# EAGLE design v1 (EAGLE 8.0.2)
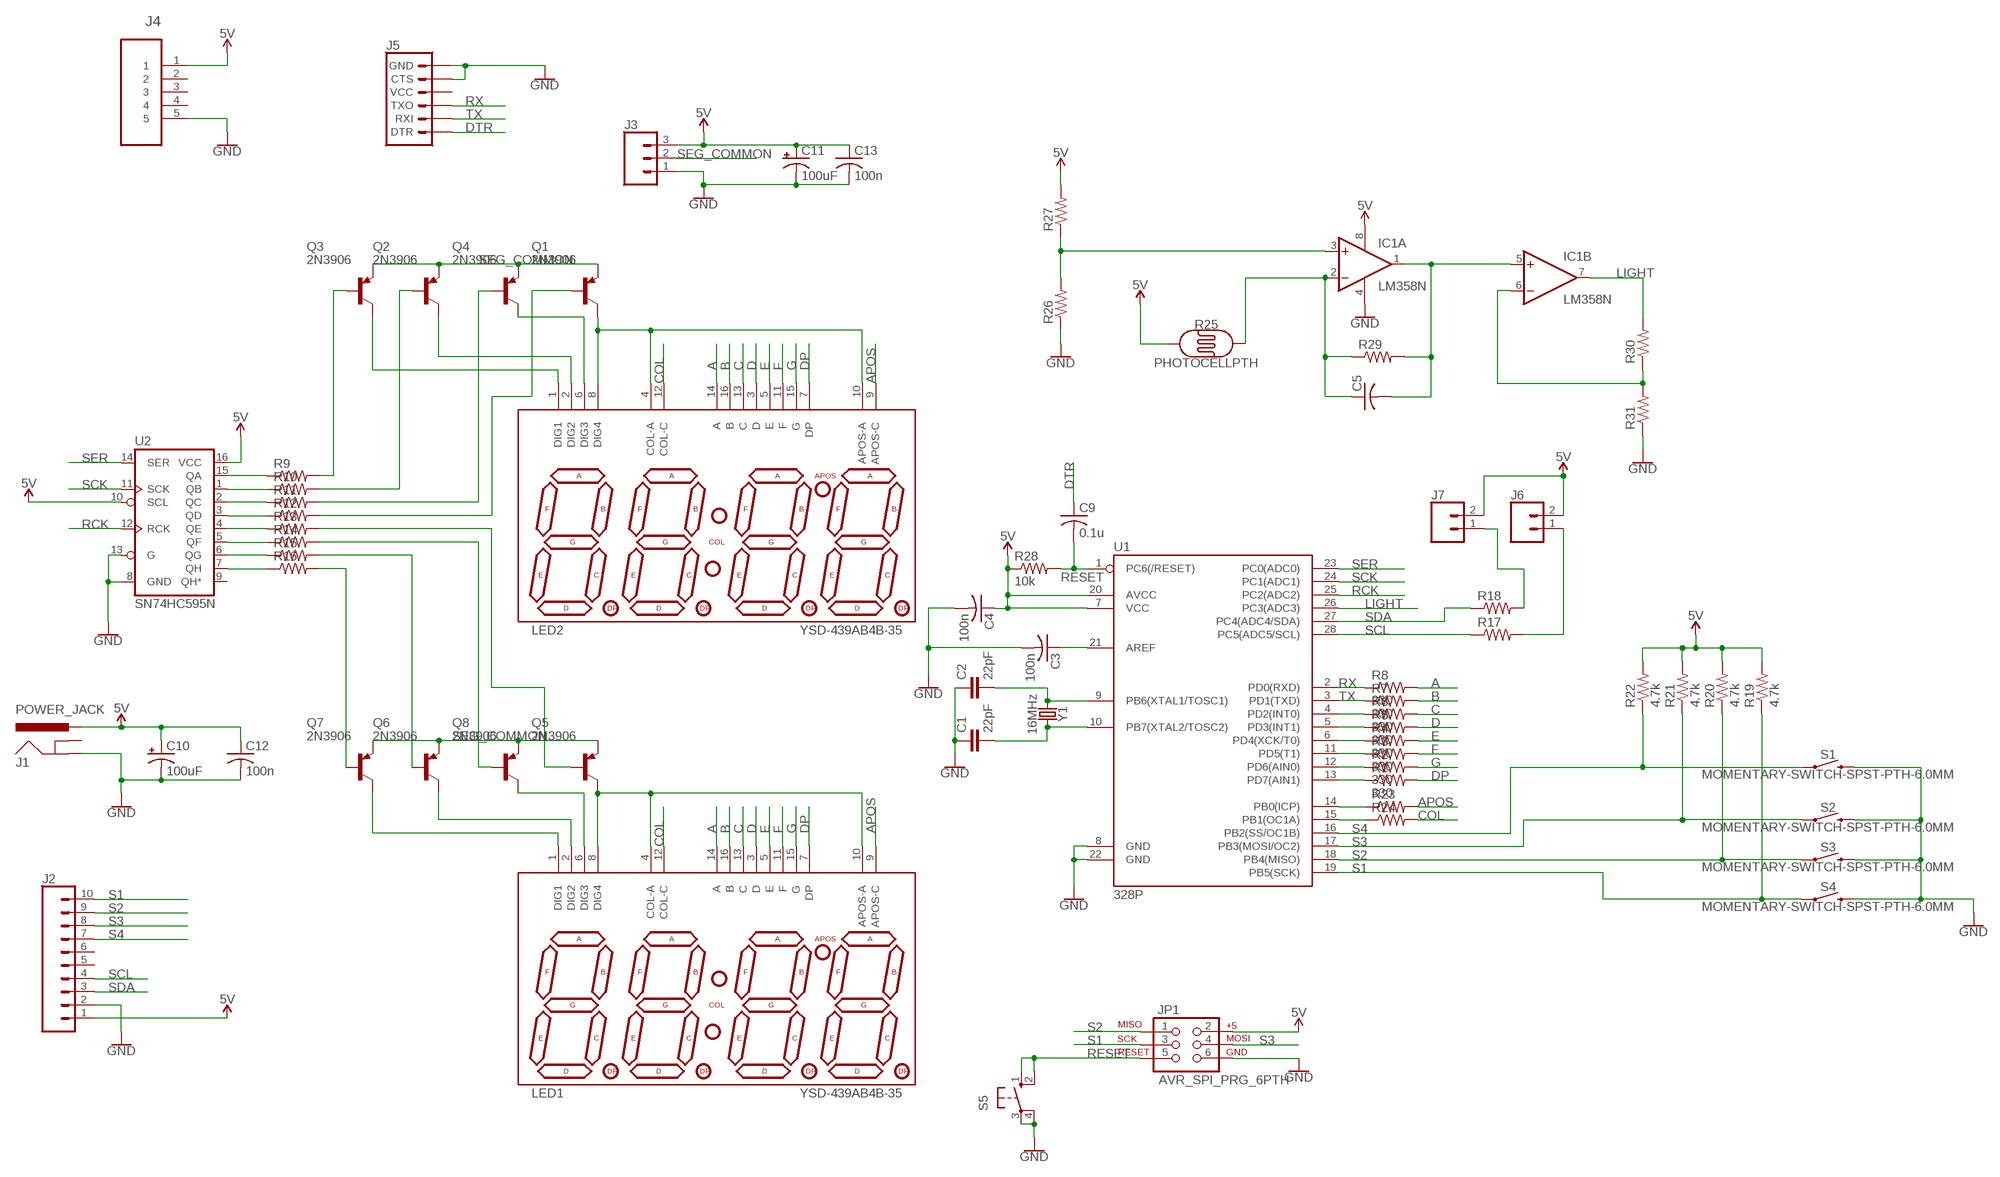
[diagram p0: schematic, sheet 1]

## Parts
C1  22pF  22PF-PTH-2.54MM-200V-5%  [CAP-PTH-2.54]
C2  22pF  22PF-PTH-2.54MM-200V-5%  [CAP-PTH-2.54]
C3  100n  C-US025-025X050  [C025-025X050]
C4  100n  C-US025-025X050  [C025-025X050]
C5  C-US025-025X050  [C025-025X050]
C9  0.1u  C-US025-025X050  [C025-025X050]
C10  100uF  100UF-POLAR-RADIAL-2.5MM-25V-20%  [CPOL-RADIAL-2.5MM-6.5MM]
C11  100uF  100UF-POLAR-RADIAL-2.5MM-25V-20%  [CPOL-RADIAL-2.5MM-6.5MM]
C12  100n  C-US025-025X050  [C025-025X050]
C13  100n  C-US025-025X050  [C025-025X050]
IC1  LM358N  [DIL08]
J1  POWER_JACK  [POWER_JACK_PTH]
J2  CONN_10"  [1X10]
J3  CONN_03  [1X03]
J4  47346-0001  [MOLEX_47346-0001]
J5  6_PIN_SERIAL_TARGET  [1X06]
J6  CONN_02  [1X02]
J7  CONN_02  [1X02]
JP1  AVR_SPI_PRG_6PTH  [2X3]
LED1  YSD-439AB4B-35  7-SEGMENT-4DIGIT-10MM-BLUE  [7-SEGMENT-4DIGIT-YOUNGSUN]
LED2  YSD-439AB4B-35  7-SEGMENT-4DIGIT-10MM-BLUE  [7-SEGMENT-4DIGIT-YOUNGSUN]
Q1  2N3906  [TO92]
Q2  2N3906  [TO92]
Q3  2N3906  [TO92]
Q4  2N3906  [TO92]
Q5  2N3906  [TO92]
Q6  2N3906  [TO92]
Q7  2N3906  [TO92]
Q8  2N3906  [TO92]
R1  330  R-US_0204/5  [0204/5]
R2  330  R-US_0204/5  [0204/5]
R3  330  R-US_0204/5  [0204/5]
R4  330  R-US_0204/5  [0204/5]
R5  330  R-US_0204/5  [0204/5]
R6  330  R-US_0204/5  [0204/5]
R7  330  R-US_0204/5  [0204/5]
R8  330  R-US_0204/5  [0204/5]
R9  R-US_0204/5  [0204/5]
R10  R-US_0204/5  [0204/5]
R11  R-US_0204/5  [0204/5]
R12  R-US_0204/5  [0204/5]
R13  R-US_0204/5  [0204/5]
R14  R-US_0204/5  [0204/5]
R15  R-US_0204/5  [0204/5]
R16  R-US_0204/5  [0204/5]
R17  R-US_0204/5  [0204/5]
R18  R-US_0204/5  [0204/5]
R19  4.7k  R-US_0204/5  [0204/5]
R20  4.7k  R-US_0204/5  [0204/5]
R21  4.7k  R-US_0204/5  [0204/5]
R22  4.7k  R-US_0204/5  [0204/5]
R23  R-US_0204/5  [0204/5]
R24  R-US_0204/5  [0204/5]
R25  PHOTOCELLPTH  [PHOTOCELL]
R26  R-US_0204/5  [0204/5]
R27  R-US_0204/5  [0204/5]
R28  10k  R-US_0204/5  [0204/5]
R29  R-US_0204/5  [0204/5]
R30  R-US_0204/5  [0204/5]
R31  R-US_0204/5  [0204/5]
S1  MOMENTARY-SWITCH-SPST-PTH-6.0MM  [TACTILE_SWITCH_PTH_6.0MM]
S2  MOMENTARY-SWITCH-SPST-PTH-6.0MM  [TACTILE_SWITCH_PTH_6.0MM]
S3  MOMENTARY-SWITCH-SPST-PTH-6.0MM  [TACTILE_SWITCH_PTH_6.0MM]
S4  MOMENTARY-SWITCH-SPST-PTH-6.0MM  [TACTILE_SWITCH_PTH_6.0MM]
S5  10-XX  [B3F-10XX]
U1  328P  ATMEGA328P_PDIP  [DIP28]
U2  SN74HC595N  74HC595N  [DIP16]
Y1  16MHz  CRYSTAL-16MHZPTH-HC49US  [HC49US]

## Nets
5V [SUPPLY]: C4.1 C10.1(+) C11.1(+) C12.1 C13.1 IC1.8(P:V+) J1.PWR J2.1 J3.3 J4.1 J6.2 J7.2 JP1.2 R19.2 R20.2 R21.2 R22.2 R25.1 R27.2 R28.1 U1.7(VCC) U1.20(AVCC) U2.10(SCL) U2.16(VCC)
A: LED1.14(A) LED2.14(A) R8.2
APOS: LED1.9(APOS-C) LED2.9(APOS-C) R23.2
B: LED1.16(B) LED2.16(B) R7.2
C: LED1.13(C) LED2.13(C) R6.2
COL: LED1.12(COL-C) LED2.12(COL-C) R24.2
D: LED1.3(D) LED2.3(D) R5.2
DP: LED1.7(DP) LED2.7(DP) R1.2
DTR: C9.1 J5.1(DTR)
E: LED1.5(E) LED2.5(E) R4.2
F: LED1.11(F) LED2.11(F) R3.2
G: LED1.15(G) LED2.15(G) R2.2
GND [SUPPLY]: C1.1 C2.1 C3.2 C4.2 C10.2(-) C11.2(-) C12.2 C13.2 IC1.4(P:V-) J1.GND J2.2 J3.1 J4.5 J5.5(CTS) J5.6(GND) JP1.6 R26.1 R31.1 S1.3 S2.3 S3.3 S4.3 S5.3(P) S5.4(P1) U1.8(GND) U1.22(GND) U2.8(GND) U2.13(G)
LIGHT: IC1.7(B:OUT) R30.2 U1.26(PC3(ADC3))
N$2: R24.1 U1.15(PB1(OC1A))
N$3: R6.1 U1.4(PD2(INT0))
N$4: R5.1 U1.5(PD3(INT1))
N$5: R4.1 U1.6(PD4(XCK/T0))
N$6: R3.1 U1.11(PD5(T1))
N$7: R2.1 U1.12(PD6(AIN0))
N$8: R1.1 U1.13(PD7(AIN1))
N$9: C2.2 U1.9(PB6(XTAL1/TOSC1)) Y1.1
N$10: C1.2 U1.10(PB7(XTAL2/TOSC2)) Y1.2
N$11: LED2.4(COL-A) LED2.8(DIG4) LED2.10(APOS-A) Q1.1(C)
N$12: LED2.6(DIG3) Q4.1(C)
N$13: LED2.2(DIG2) Q2.1(C)
N$14: LED2.1(DIG1) Q3.1(C)
N$15: LED1.4(COL-A) LED1.8(DIG4) LED1.10(APOS-A) Q5.1(C)
N$16: IC1.3(A:+IN) R26.2 R27.1
N$17: LED1.6(DIG3) Q8.1(C)
N$18: LED1.2(DIG2) Q6.1(C)
N$19: C5.1 IC1.2(A:-IN) R25.2 R29.1
N$20: LED1.1(DIG1) Q7.1(C)
N$21: Q3.2(B) R9.2
N$22: Q2.2(B) R10.2
N$23: Q4.2(B) R11.2
N$24: Q1.2(B) R12.2
N$25: Q5.2(B) R13.2
N$26: Q8.2(B) R14.2
N$27: Q6.2(B) R15.2
N$28: Q7.2(B) R16.2
N$29: R9.1 U2.15(QA)
N$30: R10.1 U2.1(QB)
N$31: R11.1 U2.2(QC)
N$32: R12.1 U2.3(QD)
N$33: R13.1 U2.4(QE)
N$34: R14.1 U2.5(QF)
N$35: R15.1 U2.6(QG)
N$36: R16.1 U2.7(QH)
N$37: C3.1 U1.21(AREF)
N$38: C5.2 IC1.1(A:OUT) IC1.5(B:+IN) R29.2
N$39: J7.1 R18.2
N$40: J6.1 R17.2
N$43: IC1.6(B:-IN) R30.1 R31.2
N$46: R23.1 U1.14(PB0(ICP))
RCK: U1.25(PC2(ADC2)) U2.12(RCK)
RESET: C9.2 JP1.5 R28.2 S5.1(S) S5.2(S1) U1.1(PC6(/RESET))
RX: J5.3(TXO) R8.1 U1.2(PD0(RXD))
S1: J2.10 JP1.3 R19.1 S4.1 U1.19(PB5(SCK))
S2: J2.9 JP1.1 R20.1 S3.1 U1.18(PB4(MISO))
S3: J2.8 JP1.4 R21.1 S2.1 U1.17(PB3(MOSI/OC2))
S4: J2.7 R22.1 S1.1 U1.16(PB2(SS/OC1B))
SCK: U1.24(PC1(ADC1)) U2.11(SCK)
SCL: J2.4 R17.1 U1.28(PC5(ADC5/SCL))
SDA: J2.3 R18.1 U1.27(PC4(ADC4/SDA))
SEG_COMMON [SUPPLY]: J3.2 Q1.3(E) Q2.3(E) Q3.3(E) Q4.3(E) Q5.3(E) Q6.3(E) Q7.3(E) Q8.3(E)
SER: U1.23(PC0(ADC0)) U2.14(SER)
TX: J5.2(RXI) R7.1 U1.3(PD1(TXD))
Unconnected: J1.GNDBREAK J2.5 J2.6 J4.2 J4.3 J4.4 J5.4(VCC) U2.9(QH*)

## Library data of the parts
C1 C2 = SparkFun-Capacitors:22PF: 22pF ceramic capacitors; PROD_ID: CAP-09128
C3-C5 C9 C12 C13 = adafruit:C-US: CAPACITOR, American symbol
C10 C11 = SparkFun-Capacitors:100UF-POLAR: 100µF polarized capacitors; PROD_ID: CAP-08439
IC1 = linear:LM358: OP AMP also LM158; LM258; LM2904 Source: http://cache.national.com/ds/LM/LM158.pdf
J1 = SparkFun-Connectors:POWER_JACK: Power Jack Connector This is the standard 5.5mm barrel jack for power. The PTH is the most common, proven, reliable, footprint. The Slot footprint only works if the mill layer is transmitted to the PCB fab house so be warned. Here are the connectors we sell at SparkFun: DC Barrel Power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; PROD_ID: CONN-08197
J2 = SparkFun-Connectors:CONN_10: Multi connection point. Often used as Generic Header-pin footprint for 0.1 inch spaced/style header connections On any of the 0.1 inch spaced packages, you can populate with these: Break Away Headers - Straight (PRT-00116) Break Away Male Headers - Right Angle (PRT-00553) Female Headers (PRT-00115)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; PROD_ID: CONN-11563
J3 = SparkFun-Connectors:CONN_03: Multi connection point. Often used as Generic Header-pin footprint for 0.1 inch spaced/style header connections On any of the 0.1 inch spaced packages, you can populate with these: Break Away Headers - Straight (PRT-00116) Break Away Male Headers - Right Angle (PRT-00553) Female Headers (PRT-00115)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
J4 = Molex-47346-0001:47346-0001: CONN RCPT 5POS MICRO USB R/A SMD; MPN: 47346-0001; OC_FARNELL: 1568026; OC_NEWARK: 47M0505; PACKAGE: 5 POS MICRO USB R/A; SUPPLIER: MOLEX
J5 = SparkFun-Connectors:6_PIN_SERIAL_TARGET: 6-pin header connection for use with the "FTDI BASIC" pinout - TARGET SIDE. Also known as "Arduino Serial Program Header". It is used to mate with our FTDI Basic serial programmers using the Arduino IDE. Note, this device has "TARGET" in the name. It is intended to be used on a design that contains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
J6 J7 = SparkFun-Connectors:CONN_02: Multi connection point. Often used as Generic Header-pin footprint for 0.1 inch spaced/style header connections
JP1 = SparkFun-Connectors:AVR_SPI_PRG_6: AVR ISP 6 Pin This is the reduced ISP connector for AVR programming. Common on Arduino. This footprint will take up less PCB space and can be used with a 10-pin to 6-pin adapter such as SKU: BOB-08508 **Special note about "TEST_POINT" package. The stop mask is on the top side, so if you want your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
LED1 LED2 = SparkFun-LED:7-SEGMENT-4DIGIT-10MM: 4 Digit 7 Segment Display This is a part for the 4-Digit 7-segment LEDs from Young Sun. Different from the Digikey LEDs, all 16 pins are used. The LONGPADS Variant is used for a test jig, but you may like it because there is more pad to solder to. If you are concerned about routing space, the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; PROD_ID: COMP-09664
Q1-Q8 = transistor-pnp:2N3906: PNP Transistor
R1-R24 R26-R31 = rcl:R-US_: RESISTOR, American symbol
R25 = SparkFun-Sensors:PHOTOCELL: Photocell (Photodetector, Photo Resistor, CdS); PROD_ID: COMP-09129; SF_ID: SEN-09088
S1-S4 = SparkFun-Switches:MOMENTARY-SWITCH-SPST: Momentary Switch (Pushbutton) - SPST; PROD_ID: SWCH-08441; SF_SKU: COM-00097
S5 = switch-omron:10-XX: OMRON SWITCH; MPN: B3F-1000; OC_FARNELL: 176432; OC_NEWARK: 36M3542
U1 = SparkFun-IC-Microcontroller:ATMEGA328P_PDIP: Atmel 328P Through hole ATMEGA328P uC used in the Arduino 32kb flash, 1k EEPROM, 2k SRAM Datasheet SparkFun Products Storefront component: AVR 28 Pin 20MHz 32K 6A/D - ATMega328P (COM-09061) SparkFun Simon Says - Through-Hole Soldering Kit (KIT-10547) SparkFun Learn to Solder - Simon Says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; PROD_ID: IC-09136
U2 = SparkFun-IC-Logic:74*595: 8-Bit Shift Register (Serial to Parallel) Datasheet SparkFun Products SparkFun Shift Register Breakout - 74HC595 (BOB-10680); PROD_ID: IC-13123
Y1 = SparkFun-Clocks:CRYSTAL-16MHZ: 16MHz Crystal; PROD_ID: XTAL-08181; SF_ID: COM-00536

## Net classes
0 default: width 0.254 mm, drill 0.356 mm, clearance 0.2 mm
1 SUPPLY: width 0.4 mm, drill 0.4 mm, clearance 0.2 mm to class 0, clearance 0.2 mm

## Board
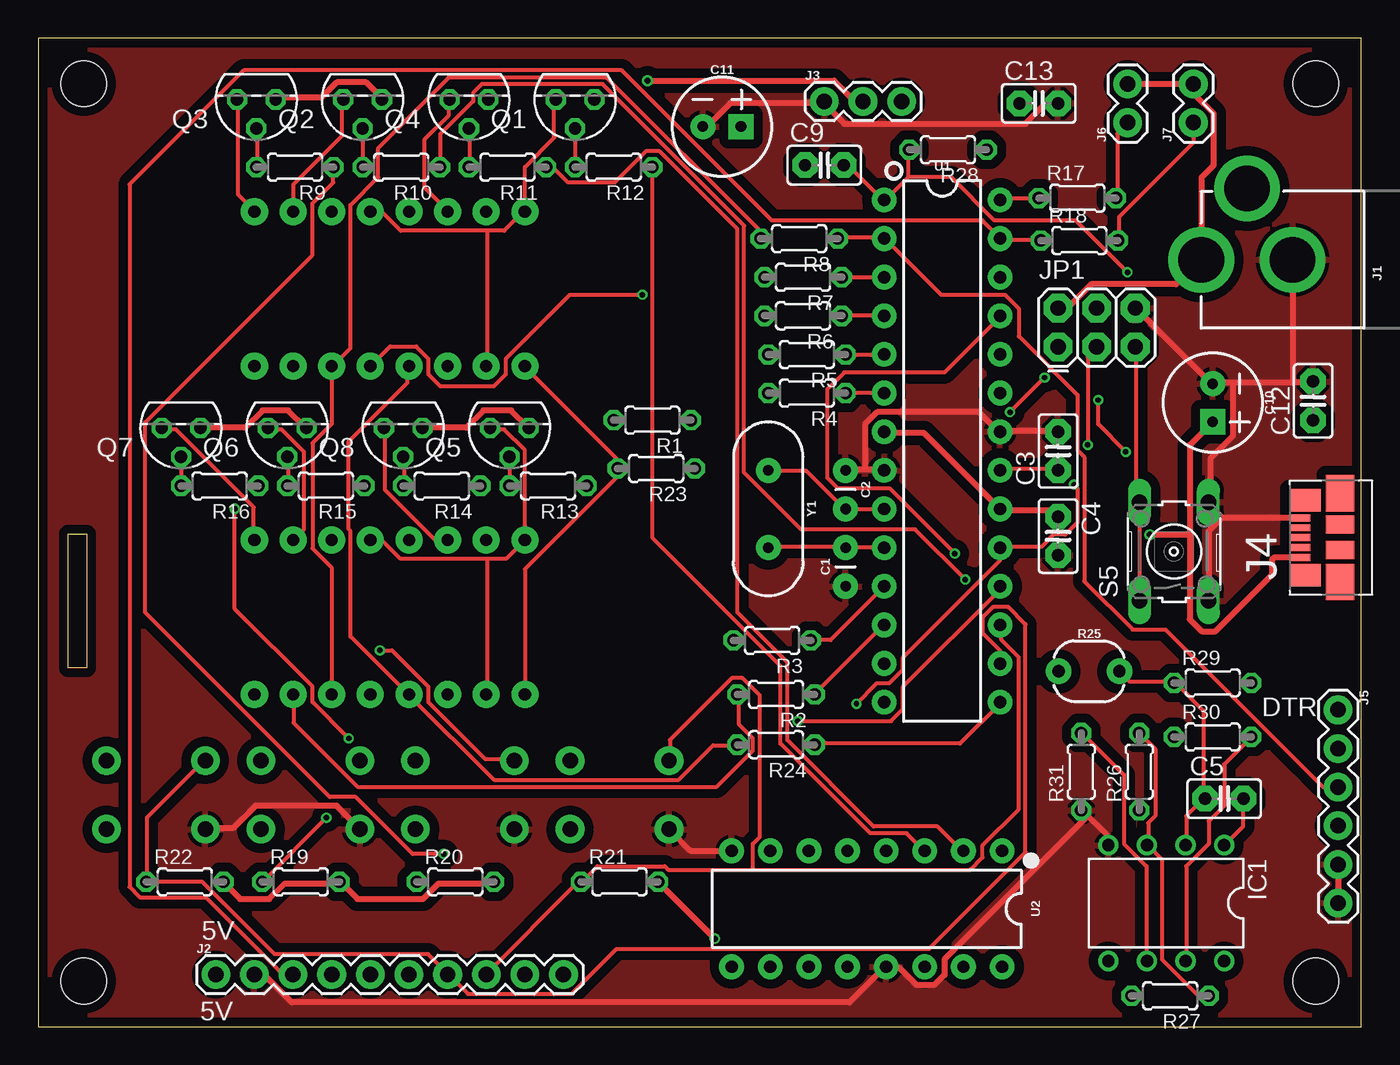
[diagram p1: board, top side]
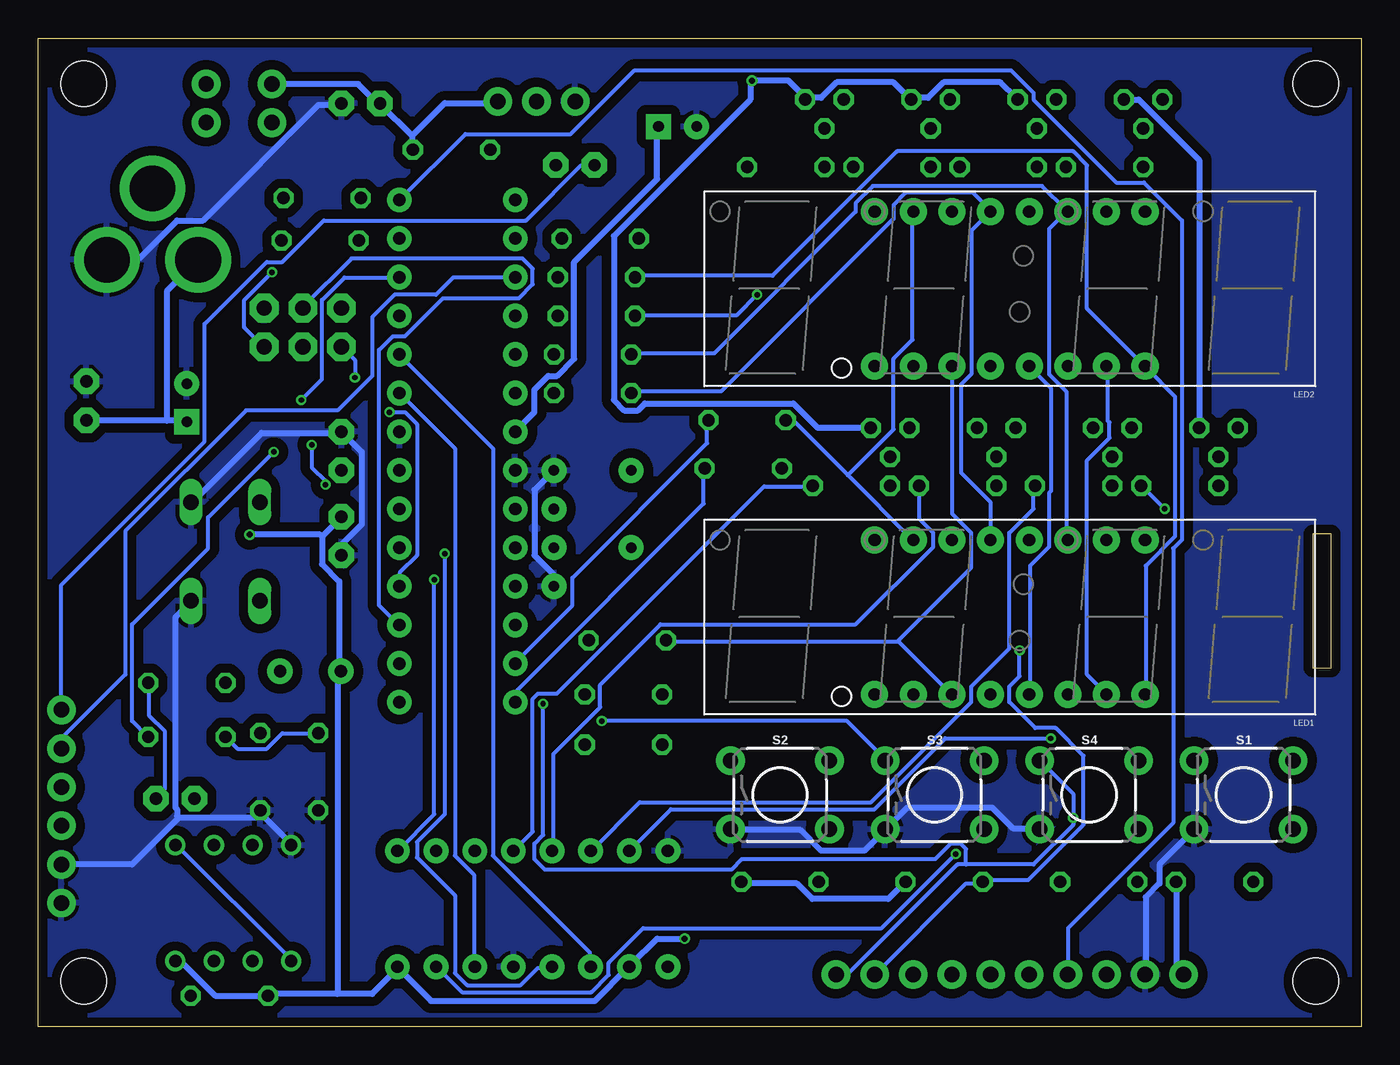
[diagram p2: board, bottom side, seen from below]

Size 87 x 65 mm. Coordinates in mm from the lower left corner, seen from the top.
Outline: 0,0 87,0 87,65 0,65 0,0
Outline: 2,32.4 3.2,32.4 3.2,23.6 2,23.6 2,32.4
Copper layers (1*16): Top 0.035mm / dielectric 1.5mm / Bottom 0.035mm
Design rules "SeeedStudio_2layer_DRU_no_angle_20140221": minimum track width 6mil, minimum drill 12mil, track to track 6mil, track to pad 6mil, pad to pad 6mil, via to via 6mil, smd to smd 0mil, copper to edge 10mil, drill to drill 10mil, minimum pad ring 10mil, minimum via ring 6mil, stop-mask expansion 2mil, vias tented up to drill 100mil, thermal gap 10mil
Holes 3 mm at 3,3 84,3 84,62 3,62
Milling: 4 lines

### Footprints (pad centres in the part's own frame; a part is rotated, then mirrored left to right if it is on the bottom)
CAP-PTH-2.54 = drill 0.7 pad 1.651: 1 -1.27,0; 2 1.27,0
C025-025X050 = drill 0.813 pad 1.676 octagon: 1 -1.27,0; 2 1.27,0
CPOL-RADIAL-2.5MM-6.5MM = drill 0.7 pad 1.651 square: 1 1.25,0 | drill 0.7 pad 1.651: 2 -1.25,0
DIL08 = drill 0.813 pad 1.27: 1 -3.81,-3.81; 2 -1.27,-3.81; 3 1.27,-3.81; 4 3.81,-3.81; 5 3.81,3.81; 6 1.27,3.81; 7 -1.27,3.81; 8 -3.81,3.81
POWER_JACK_PTH = drill 2.997 pad 4.318: GND 0,7.7; GNDBREAK 4.7,10.7; PWR 0,13.7
1X10 = drill 1.016 pad 1.88: 1 0,0; 2 2.54,0; 3 5.08,0; 4 7.62,0; 5 10.16,0; 6 12.7,0; 7 15.24,0; 8 17.78,0; 9 20.32,0; 10 22.86,0
1X03 = drill 1.016 pad 1.88: 1 0,0; 2 2.54,0; 3 5.08,0
MOLEX_47346-0001 = smd 0.45 x 1.38: 1 -1.3,0; 2 -0.65,0; 3 0,0; 4 0.65,0; 5 1.3,0 | smd 1.475 x 2.1: M1 -2.462,-0.36; M2 2.462,-0.36 | smd 2.375 x 1.9: M3 -2.913,-2.66; M6 2.913,-2.66 | smd 1.175 x 1.9: M4 -0.82,-2.66; M5 0.85,-2.66
1X06 = drill 1.016 pad 1.88: 1 0,0; 2 2.54,0; 3 5.08,0; 4 7.62,0; 5 10.16,0; 6 12.7,0
1X02 = drill 1.016 pad 1.88: 1 0,0; 2 2.54,0
2X3 = drill 1.016 pad 1.88 octagon: 1 0,0; 2 0,2.54; 3 2.54,0; 4 2.54,2.54; 5 5.08,0; 6 5.08,2.54
7-SEGMENT-4DIGIT-YOUNGSUN = drill 0.8 pad 1.778: 1 -8.89,-5.08; 2 -6.35,-5.08; 3 -3.81,-5.08; 4 -1.27,-5.08; 5 1.27,-5.08; 6 3.81,-5.08; 7 6.35,-5.08; 8 8.89,-5.08; 9 8.89,5.08; 10 6.35,5.08; 11 3.81,5.08; 12 1.27,5.08; 13 -1.27,5.08; 14 -3.81,5.08; 15 -6.35,5.08; 16 -8.89,5.08
TO92 = drill 0.813 octagon: 1 1.27,0; 2 0,1.905; 3 -1.27,0
0204/5 = drill 0.813 octagon: 1 -2.54,0; 2 2.54,0
PHOTOCELL = drill 0.8 pad 1.676: 1 -2,0; 2 2,0
TACTILE_SWITCH_PTH_6.0MM = drill 1.016 pad 1.88: 1 -3.251,2.261; 2 3.251,2.261; 3 -3.251,-2.261; 4 3.251,-2.261
B3F-10XX = drill 1.016 long: 1 -3.251,2.261; 2 3.251,2.261; 3 -3.251,-2.261; 4 3.251,-2.261
DIP28 = drill 0.813 pad 1.626: 1 -16.51,-3.81; 2 -13.97,-3.81; 3 -11.43,-3.81; 4 -8.89,-3.81; 5 -6.35,-3.81; 6 -3.81,-3.81; 7 -1.27,-3.81; 8 1.27,-3.81; 9 3.81,-3.81; 10 6.35,-3.81; 11 8.89,-3.81; 12 11.43,-3.81; 13 13.97,-3.81; 14 16.51,-3.81; 15 16.51,3.81; 16 13.97,3.81; 17 11.43,3.81; 18 8.89,3.81; 19 6.35,3.81; 20 3.81,3.81; 21 1.27,3.81; 22 -1.27,3.81; 23 -3.81,3.81; 24 -6.35,3.81; 25 -8.89,3.81; 26 -11.43,3.81; 27 -13.97,3.81; 28 -16.51,3.81
DIP16 = drill 0.813 pad 1.626: 1 -8.89,-3.81; 2 -6.35,-3.81; 3 -3.81,-3.81; 4 -1.27,-3.81; 5 1.27,-3.81; 6 3.81,-3.81; 7 6.35,-3.81; 8 8.89,-3.81; 9 8.89,3.81; 10 6.35,3.81; 11 3.81,3.81; 12 1.27,3.81; 13 -1.27,3.81; 14 -3.81,3.81; 15 -6.35,3.81; 16 -8.89,3.81
HC49US = drill 0.7 pad 1.651: 1 -2.54,0; 2 2.54,0

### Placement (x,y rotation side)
C1  53.09,30.23 90 top
C2  53.09,35.31 270 top
C3  67.06,37.85 90 top
C4  67.06,32.26 270 top
C5  77.98,14.99 0 top
C9  51.69,56.64 0 top
C10  77.22,41.02 270 top
C11  44.96,59.18 0 top
C12  83.82,41.15 90 top
C13  65.79,60.71 0 top
IC1  74.17,8.13 180 top
J1  90.17,50.42 90 top
J2  11.68,3.43 0 top
J3  51.69,60.83 0 top
J4  82.93,32.15 90 top
J5  85.47,20.83 270 top
J6  71.63,59.44 90 top
J7  75.95,59.44 90 top
JP1  67.06,44.7 0 top
LED1  23.11,26.92 180 bottom
LED2  23.11,48.51 180 bottom
Q1  35.31,60.96 180 top
Q2  21.34,60.96 180 top
Q3  14.35,60.96 180 top
Q4  28.32,60.96 180 top
Q5  30.99,39.37 180 top
Q6  16.38,39.37 180 top
Q7  9.4,39.37 180 top
Q8  24,39.37 180 top
R1  40.39,39.88 180 top
R2  48.51,21.84 180 top
R3  48.26,25.4 180 top
R4  50.55,41.66 180 top
R5  50.55,44.2 180 top
R6  50.29,46.74 180 top
R7  50.29,49.28 180 top
R8  50.04,51.82 180 top
R9  16.89,56.52 180 top
R10  23.88,56.52 180 top
R11  30.86,56.52 180 top
R12  37.85,56.52 180 top
R13  33.53,35.56 180 top
R14  26.54,35.56 180 top
R15  18.92,35.56 180 top
R16  11.94,35.56 180 top
R17  68.33,54.48 0 top
R18  68.45,51.69 0 top
R19  17.27,9.53 0 top
R20  27.43,9.53 0 top
R21  38.23,9.53 0 top
R22  9.65,9.53 0 top
R23  40.64,36.7 180 top
R24  48.51,18.54 180 top
R25  69.09,23.37 0 top
R26  72.39,16.76 90 top
R27  74.42,2.03 180 top
R28  59.82,57.66 180 top
R29  77.22,22.61 0 top
R30  77.22,19.05 0 top
R31  68.58,16.76 90 top
S1  7.75,15.24 0 bottom
S2  38.23,15.24 0 bottom
S3  28.07,15.24 0 bottom
S4  17.91,15.24 0 bottom
S5  74.68,31.24 90 top
U1  59.44,37.85 270 top
U2  54.48,7.75 180 top
Y1  48.01,34.04 270 top

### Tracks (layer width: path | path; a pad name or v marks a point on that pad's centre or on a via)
5V  (via drill 0.4)
  Top 0.4: J4.1 81.3,30.85 81.15,30.76 81.15,29.74 77.41,25.99 76.5,25.99 75.7,26.79 75.7,32.35 | J6.2 71.73,61.97 75.93,61.97 J7.2 76.05,61.86 76.05,61.29 77.29,60.04 77.29,56.64 76.5,55.84 76.5,50.62 J1.PWR 76.39,50.39 74.8,48.8 69.23,48.8 67.76,47.33 67.08,47.33 JP1.2 | 75.7,32.35 75.7,38.25 77.18,39.73 C10.1 | R22.2 12.26,9.42 13.28,8.4 15.21,8.4 16.23,9.42 19.75,9.42 R19.2 19.98,9.42 21,8.4 25.31,8.4 26.33,9.42 29.96,9.42 R20.2 | C4.1 66.97,33.6 66.62,33.94 63.33,33.94 U1.20 63.11,34.16 58.23,39.04 55.73,39.04 U1.7 | v44.49,5.79 40.86,9.42 R21.2 | v73.09,32.35 75.7,32.35
  Bottom 0.4: 62.42,58.57 62.42,57.66 R28.1 | 62.42,58.57 64.47,60.61 C13.1 64.69,60.72 65.94,61.97 71.62,61.97 J6.2 | 62.42,58.57 60.27,60.72 56.86,60.72 J3.3 | 78.54,39.84 77.29,39.84 C10.1 | 78.54,39.84 83.76,39.84 C12.1 | 78.54,39.84 78.54,48.35 76.5,50.39 J1.PWR | R22.2 12.14,9.42 12.14,3.97 11.69,3.52 J2.1 | R21.2 40.75,9.42 37.11,9.42 36.09,8.4 31.1,8.4 30.08,9.42 R20.2 | IC1.8 77.63,4.31 75.36,2.04 71.96,2.04 R27.2 71.73,2.16 67.31,2.16 | 67.31,2.16 65.03,2.16 63.45,3.75 U2.16 63.33,3.86 61.18,1.7 50.39,1.7 48.24,3.86 U2.10 48.01,4.09 46.31,5.79 v44.49,5.79 | C11.1 46.31,59.13 46.31,55.73 51.76,50.28 51.76,43.92 52.89,42.79 53.46,42.79 54.37,41.88 54.37,40.41 55.62,39.16 U1.7 | 68.33,32.23 68.33,30.42 67.19,29.28 67.19,23.38 R25.1 67.31,23.27 67.31,2.16 | 68.33,32.23 67.08,33.48 C4.1 | v73.09,32.35 68.44,32.35 68.33,32.23
A
  Top 0.254: R8.2 47.44,51.87 47.44,52.32 37.34,62.42 27.01,62.42 22.36,57.77 22.36,55.84 20.54,54.03 20.54,44.6 19.41,43.47 LED2.14 19.3,43.36 19.3,39.61 18.05,38.36 18.05,31.44 19.3,30.19 19.3,21.91 LED1.14
APOS
  Top 0.254: LED2.9 32.01,43.36 38.02,37.34 38.02,36.77 R23.2 38.02,36.66 38.02,36.09 32.01,30.08 32.01,21.91 LED1.9
B
  Bottom 0.254: R7.2 47.67,49.37 38.7,49.37 30.53,57.54 18.95,57.54 18.05,56.64 18.05,47.22 14.3,43.47 LED2.16 14.19,43.36 12.26,41.43 12.26,32.23 14.19,30.3 14.19,21.91 LED1.16
C  (via drill 0.36)
  Top 0.254: v39.73,48.12 34.96,48.12 30.76,43.92 30.76,42.9 29.96,42.11 26.45,42.11 25.65,42.9 25.65,43.92 24.86,44.72 23.15,44.72 21.91,43.47 LED2.13
  Bottom 0.254: v39.73,48.12 41.09,46.76 47.67,46.76 R6.2 | LED1.13 21.79,21.91 21.79,30.3 20.54,31.55 20.54,35.07 20.43,35.19 20.43,41.99 21.79,43.36 LED2.13
COL
  Top 0.254: R24.2 45.97,18.5 44.38,18.5 42.11,16.23 29.96,16.23 24.4,21.79 LED1.12 24.29,21.91 20.54,25.65 20.54,32.58 20.43,32.69 20.43,38.48 24.29,42.34 24.29,43.36 LED2.12
D
  Bottom 0.254: R5.2 47.9,44.27 42.56,44.27 33.26,53.57 33.26,54.14 32.12,55.27 21,55.27 19.41,53.69 LED2.3 19.41,53.57 20.54,52.44 20.54,42.9 19.41,41.77 19.41,32.01 LED1.3
DP
  Bottom 0.254: 33.77,36.26 29.51,32.01 LED1.7 | 33.77,36.26 37.34,39.84 37.8,39.84 R1.2 | 33.77,36.26 30.76,39.27 30.76,43.92 29.51,45.17 29.51,53.57 LED2.7
DTR
  Bottom 0.254: C9.1 50.51,56.64 51.3,56.64 54.93,53.01 68.21,53.01 70.94,50.28 71.96,50.28 76.05,46.19 76.05,38.48 85.47,29.06 85.47,20.88 J5.1
E
  Bottom 0.254: R4.2 47.9,41.77 42.11,41.77 30.76,53.12 30.76,54.03 29.96,54.82 25.54,54.82 24.4,53.69 LED2.5 24.4,53.57 25.65,52.32 25.65,42.9 26.33,42.22 26.33,36.43 24.4,34.5 24.4,32.01 LED1.5
F
  Bottom 0.254: 30.42,25.31 45.63,25.31 R3.2 | 30.42,25.31 27.01,21.91 LED1.11 | LED2.11 26.9,43.36 26.9,33.71 25.65,32.46 25.65,30.19 30.42,25.42 30.42,25.31
G
  Top 0.254: R2.2 46.08,21.79 46.08,19.86 46.99,18.95 46.99,18.16 44.6,15.78 21,15.78 16.8,19.98 16.8,21.79 LED1.15
  Bottom 0.254: LED2.15 16.68,43.36 16.68,39.84 16.57,39.73 16.57,38.7 18.05,37.23 18.05,23.15 16.8,21.91 LED1.15
GND
  Top 0.4: J4.5 81.2,33.45 | 81.2,33.45 | U2.8 45.51,11.58 42.9,11.58 41.54,12.94 S2.3 | S1.3 11.01,13.05 12.82,13.05 14.3,14.53 19.64,14.53 21.11,13.05 S4.3 | J5.6 85.47,8.17 85.47,10.56 J5.5 | IC1.4 70.26,12.03 70.26,12.6 68.67,14.19 R31.1 68.89,13.73 59.59,4.43 59.59,3.4 58.91,2.72 57.77,2.72 56.64,3.86 55.84,3.86 U2.13 55.62,3.86 53.34,1.59 16.68,1.59 14.87,3.4 14.3,3.4 J2.2 | C11.2 43.81,59.25 44.04,59.25 45.51,60.72 51.64,60.72 J3.1 51.76,60.61 53.01,59.36 64.92,59.36 66.17,60.61 66.97,60.61 C13.2 | 54.37,36.66 53.12,36.66 C2.1 | 54.37,36.66 55.62,36.66 U1.8 | C3.2 66.97,39.16 63.33,39.16 U1.22 63.11,39.16 61.86,40.41 55.16,40.41 54.37,39.61 54.37,36.66 | 77.86,33.48 81.04,33.48 81.2,33.45 | 77.86,33.48 76.95,34.39 S5.4 77.07,34.62 77.07,37.34 78.54,38.82 78.54,42.34 | 77.86,33.48 76.95,32.58 76.95,28.04 S5.3 | 82.51,42.34 83.76,42.34 C12.2 | 82.51,42.34 78.54,42.34 | 78.54,42.34 77.29,42.34 C10.2 77.07,42.34 72.19,47.22 JP1.6 | 82.51,42.34 82.51,50.39 J1.GND
  Bottom 0.4: J2.2 14.19,3.52 14.19,8.51 13.28,9.42 13.28,10.67 11.01,12.94 S1.3 | S4.3 21.22,13.05 22.93,13.05 24.29,14.41 29.85,14.41 31.21,13.05 S3.3 31.44,12.82 32.69,11.58 35.53,11.58 36.89,12.94 41.43,12.94 S2.3 | IC1.4 70.37,12.03 72.3,13.96 72.3,14.19 R26.1 72.3,13.73 77.75,13.73 | 77.75,13.73 80.81,10.67 J5.5 | C1.1 53.12,29.06 53.12,29.74 54.37,30.98 54.37,35.3 53.12,36.55 C2.1 | C4.2 66.97,31.1 66.97,31.78 65.72,33.03 65.72,37.8 66.97,39.04 C3.2 67.19,39.04 72.3,39.04 76.84,34.5 S5.4 | C13.2 67.08,60.61 68.55,60.61 76.16,53.01 77.86,53.01 80.36,50.51 82.4,50.51 J1.GND | 77.75,13.73 77.86,13.85 77.86,14.3 77.97,14.41 77.97,26.9 76.95,27.92 S5.3
  pour Bottom (isolate 0.61): 0,65 87,65 87,0 0,0
  pour Top (isolate 0.61): 0,65 87,65 87,0 0,0
LIGHT  (via drill 0.36)
  Top 0.254: IC1.7 75.48,4.43 75.48,10.56 76.95,12.03 76.95,13.51 77.97,14.53 77.97,17.25 79.68,18.95 R30.2 | v69.69,41.2 69.69,39.61 v71.5,37.8
  Bottom 0.254: v69.69,41.2 68.33,42.56 68.33,47.78 66.85,49.26 63.33,49.26 U1.26 | v71.5,37.8 75.82,33.48 75.82,31.44 80.81,26.45 80.81,20.09 79.79,19.07 R30.2
N$2
  Top 0.254: R24.1 51.08,18.61 60.61,18.61 63.22,21.22 U1.15
N$3
  Top 0.254: R6.1 52.89,46.76 55.62,46.76 U1.4
N$4
  Top 0.254: R5.1 53.12,44.15 55.62,44.15 U1.5
N$5
  Top 0.254: R4.1 53.12,41.65 55.62,41.65 U1.6
N$6
  Top 0.254: R3.1 50.85,25.42 52.1,25.42 55.62,28.94 U1.11
N$7
  Top 0.254: R2.1 51.08,21.91 55.62,26.45 U1.12
N$8
  Bottom 0.254: R1.1 43.02,39.84 43.02,38.36 51.87,29.51 51.87,27.69 55.62,23.95 U1.13
N$9
  Top 0.254: U1.9 55.62,34.05 53.12,34.05 C2.2 53.01,34.05 50.51,36.55 48.01,36.55 Y1.1
N$10
  Top 0.254: U1.10 55.62,31.55 53.12,31.55 C1.2 53.01,31.55 48.01,31.55 Y1.2
N$11
  Top 0.254: Q1.1 33.94,60.95 33.94,58.45 32.01,56.52 32.01,53.69 LED2.8 31.89,53.57 30.64,52.32 29.51,52.32 | 29.51,52.32 23.84,52.32 22.59,53.57 21.91,53.57 LED2.4 | 29.51,52.32 29.51,43.47 LED2.10
N$12
  Top 0.254: Q4.1 27.01,60.95 27.01,59.93 25.42,58.34 25.42,55.16 26.9,53.69 LED2.6
N$13
  Top 0.254: Q2.1 19.98,60.95 19.98,58.57 16.8,55.39 16.8,53.69 LED2.2
N$14
  Top 0.254: Q3.1 13.17,60.95 13.17,54.71 14.19,53.69 LED2.1
N$15
  Top 0.254: Q5.1 29.74,39.27 30.64,39.27 32.01,37.91 LED1.8 30.76,30.76 29.51,30.76 | 29.51,30.76 23.84,30.76 22.7,31.89 21.91,31.89 LED1.4 | 29.51,30.76 29.51,21.91 LED1.10
N$16
  Top 0.254: R26.2 72.41,19.3 73.43,18.27 73.43,13.85 72.98,13.39 72.98,12.03 IC1.3 72.98,11.92 73.89,11.01 73.89,4.43 76.27,2.04 76.95,2.04 R27.1
N$17
  Top 0.254: Q8.1 22.81,39.27 22.81,35.3 26.11,32.01 26.9,32.01 LED1.6
N$18
  Top 0.254: Q6.1 15.21,39.27 16,39.27 17.48,37.8 17.48,32.69 16.8,32.01 LED1.2
N$19
  Top 0.254: IC1.2 75.48,12.03 75.48,13.85 76.61,14.98 C5.1 76.61,15.1 76.61,20.77 74.8,22.59 R29.1 74.57,22.7 71.73,22.7 71.17,23.27 R25.2
N$20
  Top 0.254: Q7.1 8.17,39.27 9.08,39.27 14.19,34.16 14.19,32.01 LED1.1
N$21
  Top 0.254: R9.2 14.41,56.52 14.41,59.02 Q3.2
N$22
  Top 0.254: R10.2 21.34,59.02 Q2.2
N$23
  Top 0.254: R11.2 28.38,56.52 28.38,59.02 Q4.2
N$24
  Top 0.254: R12.2 35.3,56.52 35.3,59.02 Q1.2
N$25
  Top 0.254: R13.2 30.98,35.64 Q5.2
N$26
  Top 0.254: R14.2 24.06,35.64 24.06,37.45 Q8.2
N$27
  Top 0.254: R15.2 16.46,35.64 16.46,37.45 Q6.2
N$28
  Top 0.254: R16.2 9.42,35.64 9.42,37.45 Q7.2
N$29  (via drill 0.36)
  Top 0.254: v26.67,11.35 24.63,11.35 20.88,15.1 19.18,15.1 7.04,27.24 7.04,39.73 18.05,50.73 18.05,54.14 19.41,55.5 19.41,56.41 R9.1
  Bottom 0.254: v26.67,11.35 31.55,6.47 47.22,6.47 49.49,4.2 49.49,3.4 50.62,2.27 59.13,2.27 60.72,3.86 U2.15
N$30  (via drill 0.36)
  Top 0.254: v60.95,29.4 57.66,32.69 50.17,32.69 46.42,36.43 46.42,52.66 37.11,61.97 29.17,61.97 28.6,61.4 28.6,60.84 26.45,58.68 26.45,56.52 R10.1
  Bottom 0.254: v60.95,29.4 60.95,13.96 63.33,11.58 U2.1
N$31
  Top 0.254: R11.1 33.48,56.41 33.94,56.41 34.84,55.5 37.91,55.5 39.95,57.54 40.86,57.54 45.97,52.44 45.97,27.24 49.26,23.95 49.26,18.84 54.93,13.17 59.13,13.17 60.72,11.58 U2.2
N$32
  Top 0.254: R12.1 40.41,56.41 40.41,32.12 48.8,23.72 48.8,18.61 54.71,12.71 57.09,12.71 58.23,11.58 U2.3
N$33
  Bottom 0.254: R13.1 36.09,35.53 39.27,35.53 52.89,21.91 54.14,21.91 54.48,21.57 54.48,12.82 55.73,11.58 U2.4
N$34
  Bottom 0.254: R14.1 29.06,35.53 29.06,33.37 28.15,32.46 28.15,31.55 33.26,26.45 46.08,26.45 50.05,22.47 50.05,21 53.12,17.93 53.12,11.58 U2.5
N$35
  Bottom 0.254: R15.1 21.57,35.53 21.57,34.05 23.15,32.46 23.15,24.86 25.65,22.36 25.65,21.34 32.23,14.76 47.44,14.76 50.62,11.58 U2.6
N$36  (via drill 0.36)
  Top 0.254: v12.94,34.05 12.94,27.47 18.05,22.36 18.05,21.34 v20.43,18.95
  Bottom 0.254: v12.94,34.05 14.41,35.53 R16.1 | v20.43,18.95 27.35,18.95 32.01,14.3 45.4,14.3 48.12,11.58 U2.7
N$37
  Top 0.254: U1.21 63.33,36.66 66.97,36.66 C3.1
N$38
  Top 0.254: C5.2 79.22,14.98 79.22,13.17 78.09,12.03 IC1.1
  Bottom 0.254: R29.2 79.68,22.59 79.68,20.43 78.66,19.41 78.66,15.66 79.22,15.1 C5.2 | IC1.5 70.37,4.43 77.97,12.03 IC1.1
N$39
  Top 0.254: R18.2 71.05,51.76 71.05,53.23 75.93,58.11 75.93,59.36 J7.1
N$40
  Top 0.254: R17.2 70.94,54.59 70.94,58.68 71.62,59.36 J6.1
N$43
  Top 0.254: IC1.6 72.87,4.43 72.87,10.56 71.39,12.03 71.39,16.57 68.67,19.3 R31.2
  Bottom 0.254: R31.2 68.67,19.3 70.94,19.3 71.96,18.27 73.89,18.27 74.57,18.95 R30.1
N$46
  Bottom 0.254: R23.1 43.24,36.66 43.24,34.39 55.62,22.02 55.62,21.34 U1.14
RCK  (via drill 0.36)
  Top 0.254: v60.27,31.1 55.96,35.41 52.55,35.41 51.87,36.09 51.87,41.88 53.01,43.02 59.59,43.02 63.22,46.65 U1.25
  Bottom 0.254: v60.27,31.1 60.27,13.96 62.08,12.14 62.08,11.12 59.59,8.63 59.59,3.52 58.79,2.72 55.27,2.72 54.14,3.86 53.23,3.86 U2.12
RESET  (via drill 0.36)
  Top 0.254: 57.2,55.84 57.2,57.66 R28.2 | 57.2,55.84 55.73,54.37 U1.1 55.5,54.37 53.23,56.64 53.01,56.64 C9.2 | S5.1 72.41,28.04 72.41,34.39 S5.2 72.41,34.62 72.19,34.84 72.19,44.6 JP1.5 | 57.2,55.84 60.04,55.84 62.88,53.01 68.21,53.01 v71.62,49.6
  Bottom 0.254: v71.62,49.6 73.43,47.78 73.43,45.97 72.19,44.72 JP1.5
RX
  Top 0.254: R8.1 52.66,51.87 55.62,51.87 U1.2 55.73,51.76 59.36,48.12 63.56,48.12 64.47,47.22 64.47,45.4 68.33,41.54 68.33,37.91 68.78,37.45 68.78,29.28 71.96,26.11 74.11,26.11 84.44,15.78 85.47,15.78 J5.3
S1  (via drill 0.36)
  Top 0.254: v68.1,35.64 68.33,35.41 68.33,33.14 67.53,32.35 66.74,32.35 65.94,31.55 63.33,31.55 U1.19 63.22,31.44 63.22,30.64 56.86,24.29 56.86,23.49 55.96,22.59 55.16,22.59 v53.8,21.22 | v69.01,38.25 69.01,44.04 69.58,44.6 JP1.3 | v18.95,13.73 14.76,9.53 R19.1
  Bottom 0.254: v68.1,35.64 68.1,35.87 69.01,36.77 v69.01,38.25 | S4.1 21.11,17.48 18.95,15.32 v18.95,13.73 18.95,13.28 21.57,10.67 25.99,10.67 | 25.99,10.67 26.56,10.67 33.71,3.52 34.5,3.52 J2.10 | v53.8,21.22 53.8,12.6 54.37,12.03 54.37,11.01 53.69,10.33 41.43,10.33 40.75,11.01 28.04,11.01 27.01,12.03 26.33,12.03 25.99,11.69 25.99,10.67
S2  (via drill 0.36)
  Top 0.254: v66.17,42.68 v63.9,40.41 | v22.47,24.74 23.27,24.74 25.65,22.36 25.65,21.34 29.4,17.59 31.21,17.59 S3.1 | v49.94,20.09 56.07,20.09 56.86,20.88 56.86,22.36 63.22,28.71 63.22,28.94 U1.18
  Bottom 0.254: v63.9,40.41 62.88,40.41 62.08,39.61 62.08,30.98 63.22,29.85 63.22,29.06 U1.18 | v66.17,42.68 66.17,43.81 66.97,44.6 JP1.1 | J2.9 31.89,3.52 25.99,9.42 24.97,9.42 R20.1 24.86,9.65 21.91,9.65 18.27,13.28 18.27,17.82 20.09,19.64 21.45,19.64 23.15,21.34 23.15,22.36 22.47,23.04 v22.47,24.74 | v49.94,20.09 33.82,20.09 31.33,17.59 S3.1
S3
  Top 0.254: J2.8 29.51,3.52 35.41,9.42 35.64,9.42 R21.1 35.75,9.53 36.77,10.56 41.2,10.56 41.43,10.33 46.99,10.33 | 46.99,10.33 61.29,10.33 62.08,11.12 62.08,11.92 64.47,14.3 64.47,24.29 63.33,25.42 63.33,26.33 U1.17 | 46.99,10.33 46.99,12.03 47.44,12.48 47.44,21.79 46.31,22.93 45.63,22.93 41.54,18.84 41.54,17.59 S2.1
  Bottom 0.254: JP1.4 69.58,47.33 66.4,50.51 55.16,50.51 54.48,49.83 54.48,48.8 55.39,47.9 60.38,47.9 62.88,45.4 63.67,45.4 64.58,44.49 64.58,27.69 63.33,26.45 U1.17
S4
  Top 0.254: S1.1 10.9,17.48 7.15,13.73 7.15,9.53 R22.1 7.26,9.53 10.78,9.53 15.55,4.77 25.65,4.77 26.9,3.52 J2.7 27.01,3.4 28.26,2.16 35.07,2.16 38.02,5.11 58.57,5.11 64.92,11.46 64.92,26.45 63.79,27.58 62.77,27.58 62.08,26.9 62.08,25.88 63.22,24.74 63.22,23.95 U1.16
SCK
  Bottom 0.254: U2.11 50.73,3.97 50.73,4.88 57.09,11.24 57.09,38.02 63.22,44.15 U1.24
SCL
  Top 0.254: R17.1 65.72,54.48 63.45,54.48 63.33,54.37 U1.28
  Bottom 0.254: J2.4 19.3,3.52 19.3,6.47 12.37,13.39 12.37,31.44 11.8,32.01 11.8,53.01 14.3,55.5 16.12,55.5 21.57,60.95 21.57,61.4 23.04,62.88 47.78,62.88 51.98,58.68 58.91,58.68 63.22,54.37 U1.28
SDA
  Top 0.254: R18.1 65.83,51.76 63.33,51.76 U1.27 63.22,51.87 62.08,53.01 48.24,53.01 38.36,62.88 13.51,62.88 6.02,55.39 6.02,9.19 6.7,8.51 11.01,8.51 16,3.52 16.68,3.52 J2.3
SEG_COMMON  (via drill 0.4)
  Top 0.4: Q8.3 25.31,39.38 28.15,39.38 29.28,40.52 31.1,40.52 32.23,39.38 Q5.3 | Q7.3 10.67,39.38 13.62,39.38 14.76,40.52 16.46,40.52 17.59,39.38 Q6.3 | Q3.3 15.66,61.06 18.61,61.06 19.64,62.08 21.57,62.08 22.59,61.06 Q2.3 | v40.07,62.2 52.32,62.2 53.69,60.84 54.14,60.84 J3.2
  Bottom 0.4: Q2.3 22.7,61.06 23.72,62.08 27.47,62.08 28.49,61.06 29.51,61.06 Q4.3 29.74,61.06 30.76,62.08 34.5,62.08 35.53,61.06 36.55,61.06 Q1.3 36.66,61.18 37.68,62.2 v40.07,62.2 40.18,62.08 40.18,60.95 49.15,51.98 49.15,41.2 48.47,40.52 47.56,40.52 47.1,40.97 37.34,40.97 35.75,39.38 32.35,39.38 Q5.3 | Q7.3 10.67,39.38 10.67,56.98 14.64,60.95 15.55,60.95 Q3.3
SER
  Bottom 0.254: U2.14 58.34,3.97 58.34,9.99 59.59,11.24 59.59,38.02 63.22,41.65 U1.23
TX
  Top 0.254: R7.1 52.89,49.26 55.62,49.26 U1.3
  Bottom 0.254: J5.2 85.47,18.39 85.47,18.95 81.27,23.15 81.27,32.58 73.32,40.52 67.31,40.52 65.03,42.79 65.03,46.65 63.56,48.12 60.84,48.12 59.7,49.26 55.73,49.26 U1.3

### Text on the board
tNames: DTR | 5V | 5V

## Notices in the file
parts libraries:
SparkFun-LED: Licensing: Creative Commons ShareAlike 4.0 International - https://creativecommons.org/licenses/by-sa/4.0
